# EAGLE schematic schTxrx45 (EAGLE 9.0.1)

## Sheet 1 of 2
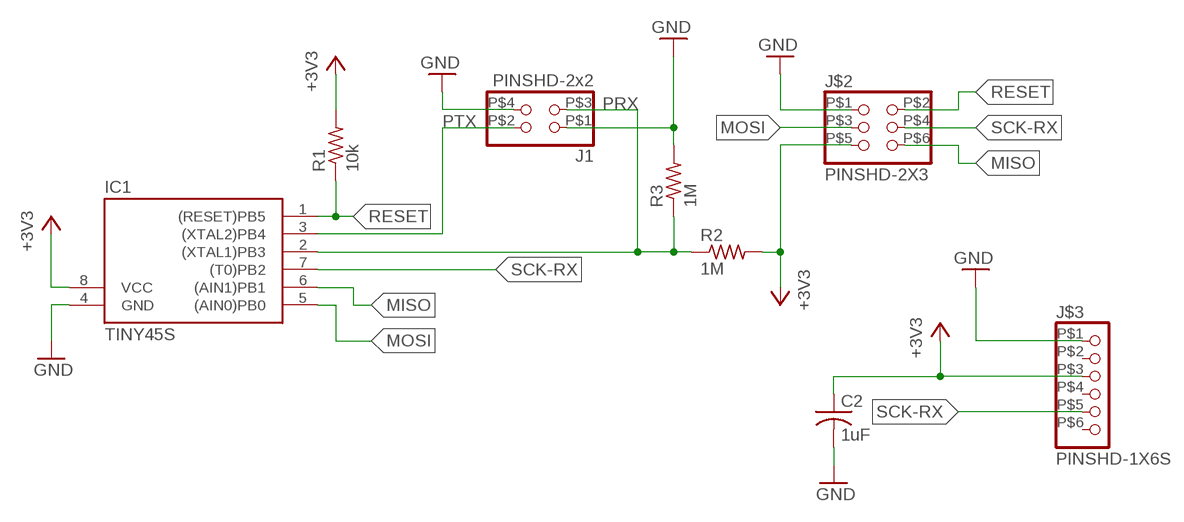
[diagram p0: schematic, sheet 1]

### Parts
C2  1uF  C-USC0805  [C0805]
IC1  TINY45S  [SOIC8]
J1  PINSHD-2x2  PINSHD-2X2  [2X02]
J$2  PINSHD-2X3  [2X03]
J$3  PINSHD-1X6S  [1X06]
R1  10k  R-US_R0805W  [R0805W]
R2  1M  R-US_R0805W  [R0805W]
R3  1M  R-US_R0805W  [R0805W]

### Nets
+3V3: C2.1 IC1.8(VCC) J$2.P$5 J$3.P$3 R1.2 R2.2
GND: C2.2 IC1.4(GND) J1.P$1 J1.P$4 J$2.P$1 J$3.P$1 R3.2
MISO: IC1.6((AIN1)PB1) J$2.P$6
MOSI: IC1.5((AIN0)PB0) J$2.P$3
PRX: IC1.2((XTAL1)PB3) J1.P$3 R2.1 R3.1
PTX: IC1.3((XTAL2)PB4) J1.P$2
RESET: IC1.1((RESET)PB5) J$2.P$2 R1.1
SCK-RX: IC1.7((T0)PB2) J$2.P$4 J$3.P$5
Unconnected: J$3.P$2 J$3.P$4 J$3.P$6

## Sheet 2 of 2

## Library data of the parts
C2 = resistor:C-US: CAPACITOR, American symbol
IC1 = atmel_mcu:TINY45*: MICROCONTROLLER 4K bytes FLASH
J1 = pinhead_smd:PINSHD-2X2
J$2 = pinhead_smd:PINSHD-2X3
J$3 = pinhead_smd:PINSHD-1X6
R1-R3 = resistor:R-US_: RESISTOR, American symbol

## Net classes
0 default: width 0.254 mm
